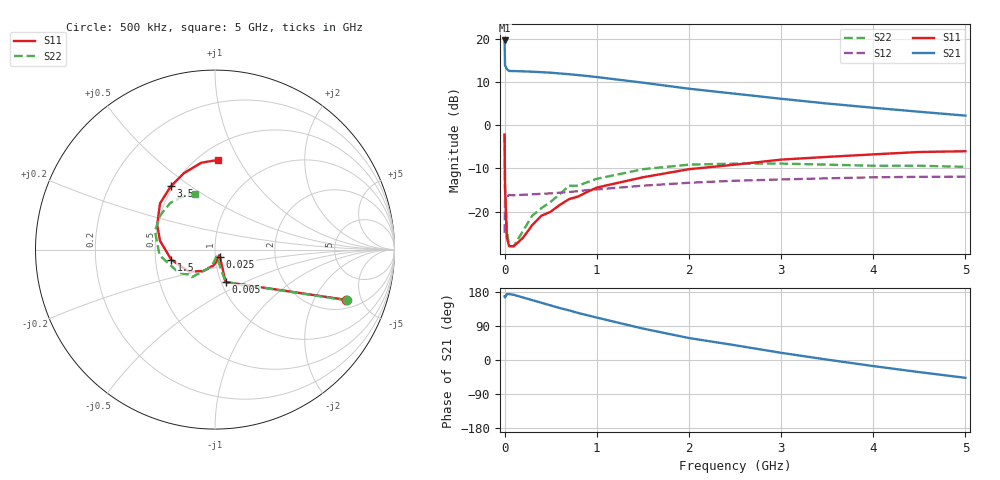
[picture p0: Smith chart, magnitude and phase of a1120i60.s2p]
!  MSA-1120 S AND NOISE PARAMETERS
!  Id=60mA  LAST UPDATED 07-27-92
# ghz s ma r 50
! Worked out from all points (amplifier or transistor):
!   22 points, 500 kHz to 5 GHz, reference 50 ohm
!   highest |S21| = 19.6 dB at 500 kHz (marker M1)
!   |S21| within 3 dB of that: start of sweep to 2.844 MHz
!   unconditionally stable (mu >= 1): 7.2 MHz to 902.1 MHz; 3.223 GHz to end of sweep
!   at 50 MHz: K = 1.08, MAG = 12.6 dB, |S12| = -16.1 dB
!   at 800 MHz: K = 1.02, MAG = 12.6 dB, |S12| = -15.2 dB
!   at 5 GHz: K = 1.11, MAG = 5.1 dB, |S12| = -11.9 dB
!   lowest NFmin = 3.30 dB at 100 MHz
!   S11 on the Smith chart (normalised r, x): 500 kHz: 2.58, -3.68; 5 MHz: 1.05, -0.39; 25 MHz: 1.05, -0.09; 1.5 GHz: 0.60, -0.07; 3.5 GHz: 0.49, +0.42; 5 GHz: 0.62, +0.82
0.0005  0.78 -21.0  9.53 168.0  0.057 50.0  0.79 -21.0
0.005  0.19 -72.0  4.91 165.0  0.144 11.0  0.19 -72.0
0.025  0.05 -56.0  4.44 174.0  0.149 3.0  0.06 -75.0
0.05  0.04 -52.0  4.23 174.0  0.156 2.0  0.04 -79.0
0.1  0.04 -56.0  4.22 172.0  0.155 1.0  0.04 -78.0
0.2  0.05 -72.0  4.19 165.0  0.157 1.0  0.06 -91.0
0.3  0.07 -84.0  4.15 158.0  0.159 2.0  0.09 -101.0
0.4  0.09 -96.0  4.1 151.0  0.161 2.0  0.11 -109.0
0.5  0.1 -105.0  4.04 144.0  0.163 3.0  0.13 -117.0
0.6  0.12 -113.0  3.96 137.0  0.166 3.0  0.16 -124.0
0.7  0.14 -120.0  3.88 131.0  0.169 2.0  0.2 -130.0
0.8  0.15 -127.0  3.79 124.0  0.173 3.0  0.2 -136.0
0.9  0.17 -134.0  3.7 118.0  0.178 1.0  0.22 -142.0
1  0.19 -140.0  3.6 112.0  0.181 2.0  0.24 -148.0
1.5  0.25 -167.0  3.1 83.0  0.2 -3.0  0.31 -174.0
2  0.31 171.0  2.64 58.0  0.216 -10.0  0.35 163.0
2.5  0.35 157.0  2.31 39.0  0.228 -16.0  0.36 148.0
3  0.4 140.0  2.02 19.0  0.236 -23.0  0.36 134.0
3.5  0.43 125.0  1.78 1.0  0.243 -30.0  0.35 125.0
4  0.46 112.0  1.59 -16.0  0.25 -38.0  0.34 118.0
4.5  0.49 99.0  1.43 -32.0  0.253 -46.0  0.34 113.0
5  0.5 88.0  1.29 -47.0  0.254 -53.0  0.33 110.0
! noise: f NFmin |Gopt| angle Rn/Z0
0.1  3.3  0.02  19  0.43
0.5  3.5  0.03  102  0.42
1  4  0.07  150  0.41
2  4.6  0.17  -160  0.41
